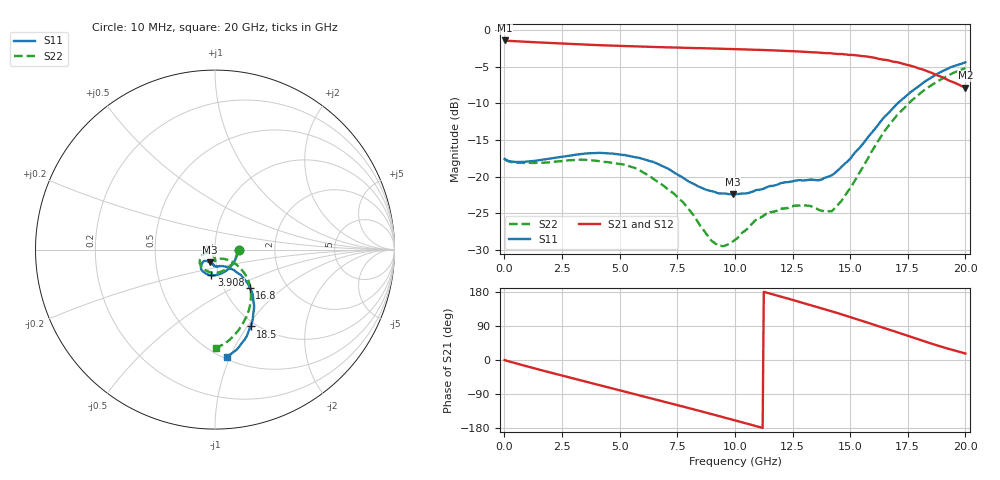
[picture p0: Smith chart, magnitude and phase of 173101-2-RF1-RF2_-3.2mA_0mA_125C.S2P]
!  2-Port S-parameters saved by WinCal
! VAR MeasName=S-Parameters (CALIBRATED_DATA) read from VNA (N5242A)
! VAR MeasDate=2017-7-20 10:59:09
! VAR NAME=173101-2-RF1-RF2_-3.2mA_0mA_125C
! VAR FILENAME=173101-2-RF1-RF2_-3.2mA_0mA_125C.S2P
! VAR DATE=2017-7-20 10:59:09
! VAR PHYS_PORTS=1,2
# Hz S DB R 50
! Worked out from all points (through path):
!   401 points, 10 MHz to 20 GHz, reference 50 ohm
!   highest |S21| = -1.41 dB at 10 MHz (marker M1); lowest = -7.9 dB at 20 GHz (marker M2)
!   group delay of S21, straight-line fit = 47.1 ps
!   lowest |S11| = -22.4 dB at 9.905 GHz (marker M3), VSWR 1.16, Z = 46.9 - j6.66 ohm
!   |S11| at or under -10 dB: start of sweep to 17.06 GHz
!   |S22| runs from -29.5 to -5.2 dB; largest |S21 - S12| = 0.0041
!   S11 on the Smith chart (normalised r, x): 10 MHz: 1.30, -0.01; 3.908 GHz: 0.92, -0.27; 16.8 GHz: 1.32, -0.61; 18.5 GHz: 0.94, -1.04; 20 GHz: 0.52, -0.97
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1e7  -17.58 -1.0  -1.41 -0.2  -1.41 -0.2  -17.60 -0.8
1.559225e9  -17.74 -48.9  -1.69 -26.2  -1.69 -26.2  -18.12 -50.9
3.358325e9  -16.91 -89.4  -1.97 -54.5  -1.97 -54.5  -17.68 -95.9
3.90805e9  -16.79 -98.3  -2.04 -63.0  -2.04 -63.0  -17.81 -106.7
5.357325e9  -17.13 -119.3  -2.20 -85.5  -2.21 -85.5  -18.52 -132.9
6.70665e9  -18.33 -129.9  -2.32 -106.6  -2.30 -106.5  -20.83 -150.4
7.756125e9  -20.16 -134.2  -2.41 -123.0  -2.41 -123.0  -23.53 -159.1
9.055475e9  -22.02 -125.5  -2.50 -143.8  -2.50 -143.8  -28.93 -144.1
9.455275e9  -22.30 -118.9  -2.55 -150.3  -2.54 -150.3  -29.50 -127.7
9.90505e9  -22.43 -111.0  -2.59 -157.7  -2.59 -157.8  -28.87 -110.4
1.0005e10  -22.40 -109.7  -2.60 -159.3  -2.60 -159.4  -28.64 -107.5
1.095452e10  -21.82 -98.9  -2.69 -175.0  -2.69 -175.0  -25.76 -89.6
1.165418e10  -21.26 -95.0  -2.76 173.1  -2.77 173.1  -24.78 -89.8
1.335332e10  -20.39 -80.4  -3.02 143.7  -3.00 143.7  -24.09 -87.6
1.410295e10  -19.98 -66.0  -3.15 130.2  -3.17 130.1  -24.77 -64.9
1.445278e10  -19.17 -60.0  -3.26 123.8  -3.25 123.9  -23.92 -53.7
1.570215e10  -14.91 -46.2  -3.60 99.7  -3.63 99.8  -17.88 -34.8
1.670165e10  -11.19 -46.7  -4.16 79.9  -4.19 79.6  -12.92 -40.1
1.68016e10  -10.87 -47.6  -4.26 77.9  -4.26 78.1  -12.52 -41.4
1.775112e10  -8.17 -56.2  -4.98 58.7  -4.99 58.7  -9.41 -53.9
1.850075e10  -6.53 -65.2  -5.79 43.7  -5.82 43.7  -7.57 -65.8
2e10  -4.40 -83.7  -7.86 17.1  -7.90 17.5  -5.19 -89.4
